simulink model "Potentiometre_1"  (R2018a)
settings: Solver=FixedStepAuto  StartTime=0.0  StopTime=inf  RelTol=1e-3  EnableMultiTasking=on
libraries: arduinolib x1

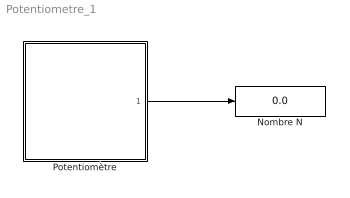
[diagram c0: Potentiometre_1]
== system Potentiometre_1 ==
  Nombre N : Display
  Potentiomètre : Subsystem
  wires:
  Potentiomètre/1(Out1) -> Nombre N/1

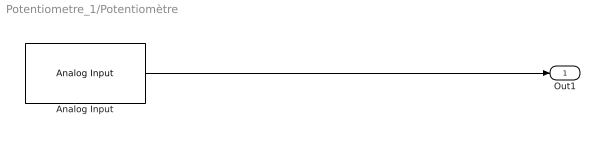
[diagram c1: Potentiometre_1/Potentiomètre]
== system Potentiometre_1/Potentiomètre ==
  Analog Input : arduinolib/Analog Input  pinNumber=5  ReadResultsOnly=off  ConversionTriggerSource=Software  ExternalTriggerType=uint32(0)  OutputDataType=uint16  EnableConversionCompleteNotify=off  EnableOuputStatus=off  SampleTime=0.01  blockPlatform=arduino
  Out1 : Outport
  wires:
  Analog Input/1 -> Out1/1
